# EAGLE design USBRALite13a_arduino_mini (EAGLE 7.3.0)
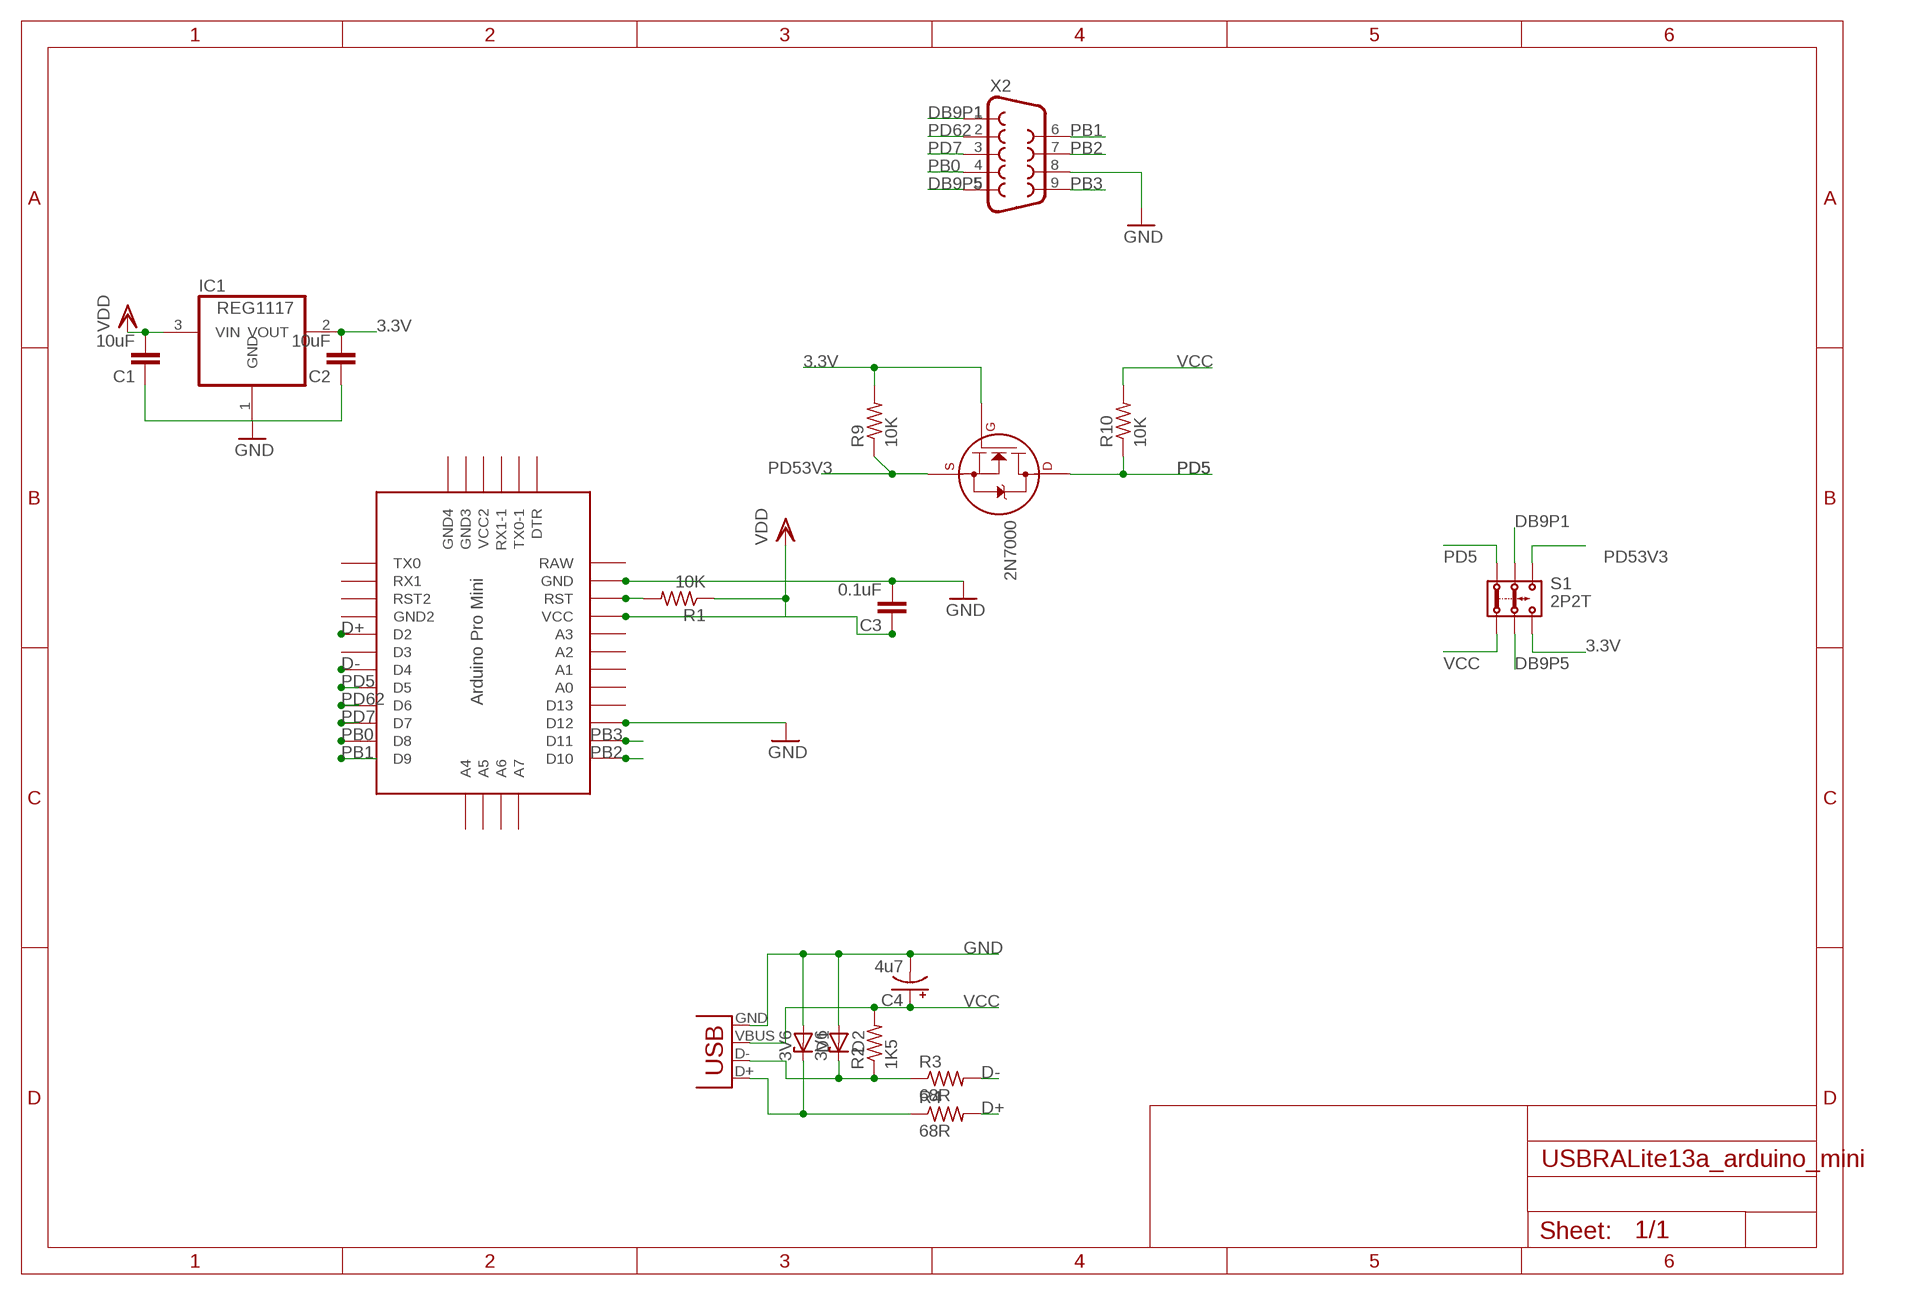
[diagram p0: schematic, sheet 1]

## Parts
2N7000  2N7000_TO92  [TO-92]
C1  10uF  C-EU050-024X044  [C050-024X044]
C2  10uF  C-EU050-024X044  [C050-024X044]
C3  0.1uF  C-EU050-024X044  [C050-024X044]
C4  4u7  CPOL-USE2.5-6  [E2,5-6]
D1  3V6  ZENER-DIODEZD-5  [ZDIO-5]
D2  3V6  ZENER-DIODEZD-5  [ZDIO-5]
IC1  REG1117  [SOT223]
R1  10K  R-US_0207/10  [0207/10]
R2  1K5  R-US_0207/10  [0207/10]
R3  68R  R-US_0207/10  [0207/10]
R4  68R  R-US_0207/10  [0207/10]
R9  10K  R-US_0207/10  [0207/10]
R10  10K  R-US_0207/10  [0207/10]
S1  2P2T  [2P2T]
U$1  PRO-MINI  [PRO-MINI]
X1  USBPTH  [USB-B-PTH]
X2  DB9MALE  [DB9_MALE]

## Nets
3.3V: 2N7000.2(G) C2.2 IC1.2(VOUT) R9.2 S1.3.2
D+: R4.2 U$1.D2
D-: R3.2 U$1.D4
DB9P1: S1.2.1 X2.1
DB9P5: S1.2.2 X2.5
GND: C1.1 C2.1 C3.2 C4.- D1.A D2.A IC1.1(GND) U$1.D12 U$1.GND X1.GND X2.8
N$1: R1.2 U$1.RST
N$8: D1.C R4.1 X1.D+
N$9: D2.C R2.1 R3.1 X1.D-
PB0: U$1.D8 X2.4
PB1: U$1.D9 X2.6
PB2: U$1.D10 X2.7
PB3: U$1.D11 X2.9
PD5: 2N7000.3(D) R10.1 S1.1.1 U$1.D5
PD7: U$1.D7 X2.3
PD53V3: 2N7000.1(S) R9.1 S1.3.1
PD62: U$1.D6 X2.2
VCC: C3.1 C4.+ R1.1 R2.2 R10.2 S1.1.2 X1.VBUS ; supply symbol labelled VDD
VDD: C1.2 IC1.3(VIN)
Unconnected: U$1.A0 U$1.A1 U$1.A2 U$1.A3 U$1.A4 U$1.A5 U$1.A6 U$1.A7 U$1.D3 U$1.D13 U$1.DTR U$1.GND1(GND2) U$1.GND2(GND4) U$1.GND3 U$1.RST1(RST2) U$1.RX1 U$1.RX1-1 U$1.TX0 U$1.TX0-1 U$1.VCC U$1.VCC1(VCC2)

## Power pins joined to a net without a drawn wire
RAW: U$1.RAW

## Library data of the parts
2N7000 = transistors:2N700*: 2N7000, 2N7002, NDS7002A N-channel enhancement mode MOSFET
C1-C3 = rcl:C-EU: CAPACITOR, European symbol
C4 = adafruit:CPOL-US: POLARIZED CAPACITOR, American symbol
D1 D2 = diode:ZENER-DIODE: Z-Diode
IC1 = burr-brown:REG1117: 800mA and 1A Low Dropout (LDO) Positive Regulator 1.8V, 2.5V, 2.85V, 3.3V, 5V, and Adj; MPN: REG1117; OC_FARNELL: 1097566; OC_NEWARK: 14P6981
R1-R4 R9 R10 = adafruit:R-US_: RESISTOR, American symbol
S1 = Itead_BP_110825:2P2T: BAS011
U$1 = Arduino-clone:PRO-MINI: Arduion Pro Mini Clone V1.0 www.betemcu.cu
X1 = SparkFun:USB: USB Connectors USB-B-PTH is fully proven SKU : PRT-00139 USB-miniB is fully proven SKU : PRT-00587 USB-A-PCB is untested. USB-A-H is throughly reviewed, but untested. Spark Fun Electronics SKU : PRT-00437 USB-B-SMT is throughly reviewed, but untested. Needs silkscreen touching up. USB-A-S has not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
X2 = SparkFun:DB9: DB9 Connector Standard DB9 (D-Sub 9) serial connector. Can be used for CAN bus as well as RS485 and RS232. Footprint production proven. Spark Fun Electronics SKU : PRT-00429

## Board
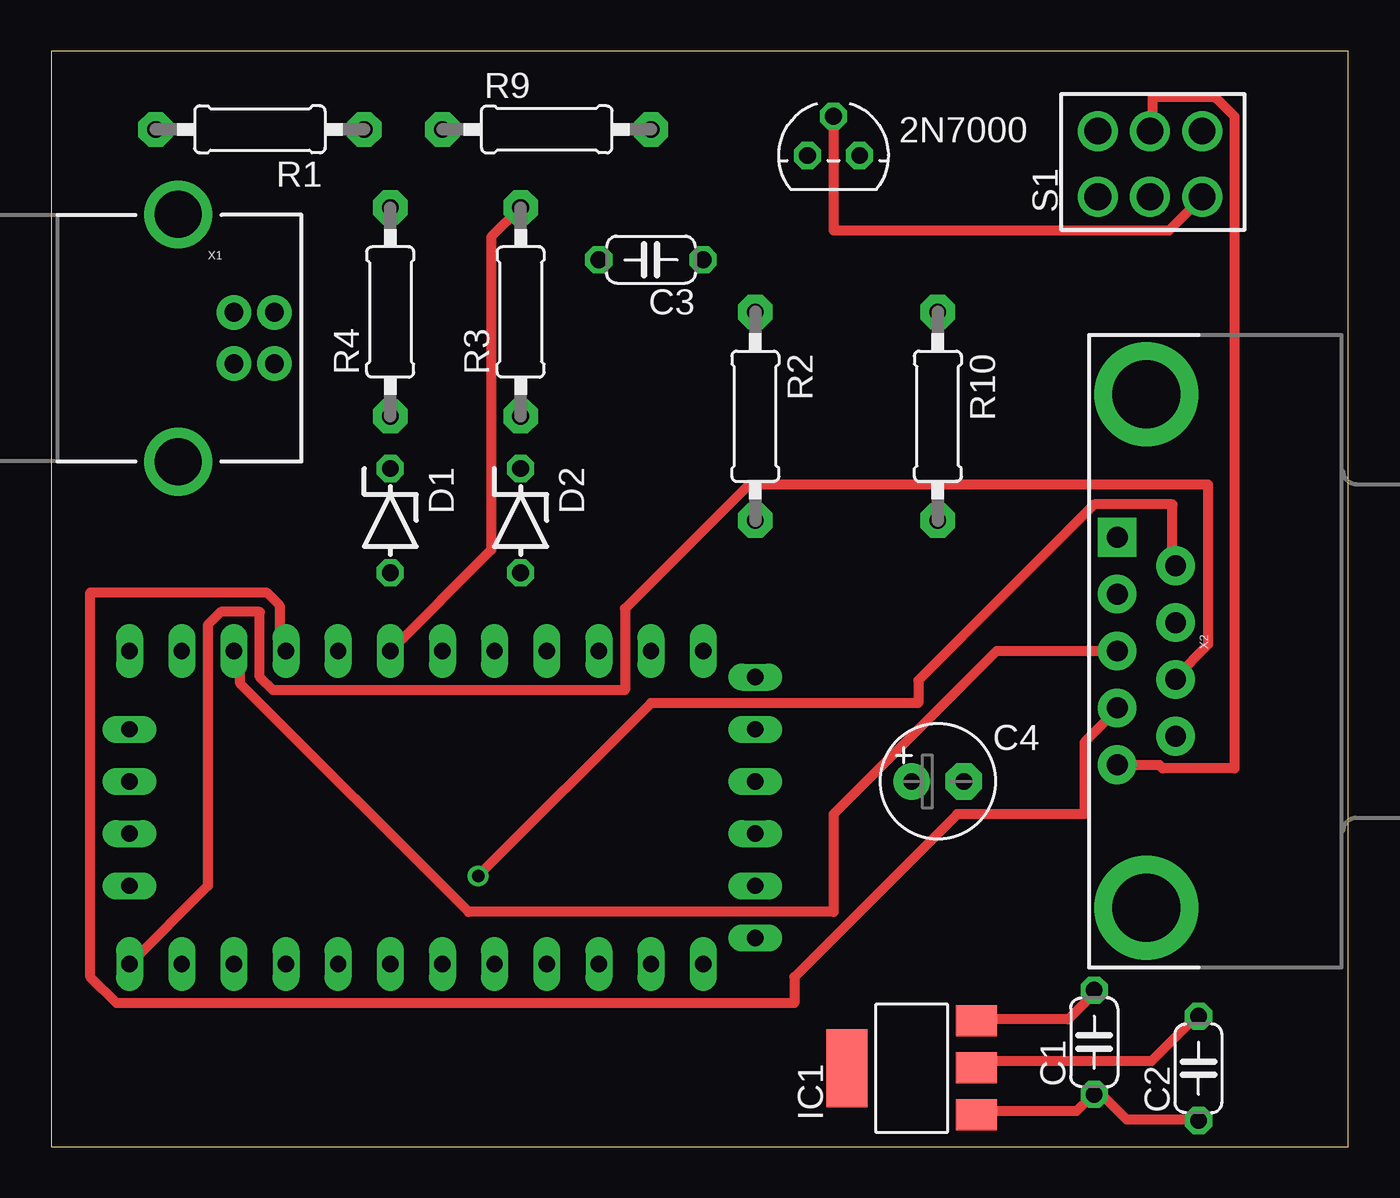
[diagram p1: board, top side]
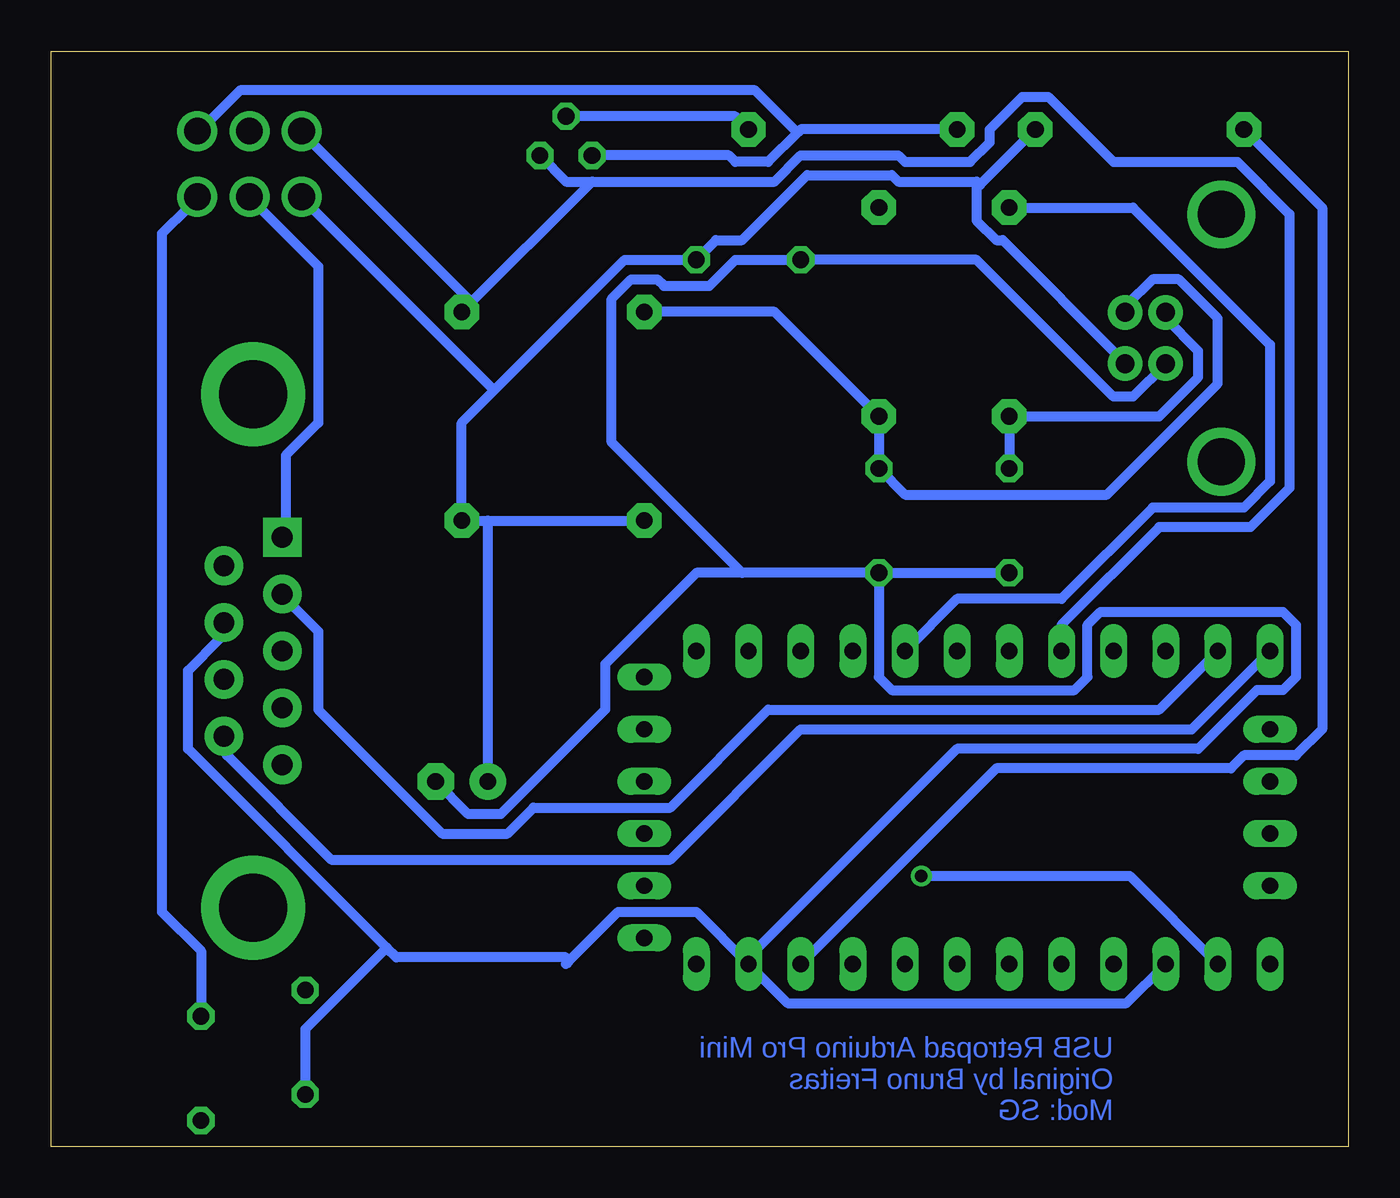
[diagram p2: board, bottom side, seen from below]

Size 63.17 x 53.33 mm. Coordinates in mm from the lower left corner, seen from the top.
Outline: 0,0 63.17,0 63.17,53.33 0,53.33 0,0
Copper layers (1*16): Top 0.035mm / dielectric 1.5mm / Bottom 0.035mm
Design rules "default *": minimum track width 19mil, minimum drill 24mil, track to track 13mil, track to pad 13mil, pad to pad 13mil, via to via 13mil, smd to smd 13mil, copper to edge 40mil, drill to drill 8mil, minimum pad ring 10mil, minimum via ring 8mil, stop-mask expansion 4mil, vias tented up to drill 0mil, thermal gap 10mil

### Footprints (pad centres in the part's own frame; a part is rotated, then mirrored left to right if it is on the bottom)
TO-92 = drill 0.813 octagon: 1 -1.27,0; 2 0,1.905; 3 1.27,0
C050-024X044 = drill 0.813 octagon: 1 -2.54,0; 2 2.54,0
E2,5-6 = drill 0.813 pad 1.778: + -1.27,0 | drill 0.813 pad 1.778 octagon: - 1.27,0
ZDIO-5 = drill 0.813 octagon: A 2.54,0; C -2.54,0
SOT223 = smd 1.499 x 2.007: 1 -2.261,-3.15; 2 0.025,-3.15; 3 2.311,-3.15 | smd 3.81 x 2.007: 4 0,3.15
0207/10 = drill 0.813 pad 1.676 octagon: 1 -5.08,0; 2 5.08,0
2P2T = drill 1.3 pad 1.93: 1.1 -3.635,-0.085; 1.2 -3.635,-3.285; 2.1 -1.095,-0.085; 2.2 -1.095,-3.285; 3.1 1.445,-0.085; 3.2 1.445,-3.285
PRO-MINI = drill 0.8 long: A0 8.89,8.89; A1 8.89,11.43; A2 8.89,13.97; A3 8.89,16.51; A4 -2.54,-1.27; A5 0,-1.27; A6 2.54,-1.27; A7 5.08,-1.27; D2 -6.35,16.51; D3 -6.35,13.97; D4 -6.35,11.43; D5 -6.35,8.89; D6 -6.35,6.35; D7 -6.35,3.81; D8 -6.35,1.27; D9 -6.35,-1.27; D10 8.89,-1.27; D11 8.89,1.27; D12 8.89,3.81; D13 8.89,6.35; DTR 7.62,29.21; GND 8.89,24.13; GND1 -6.35,19.05; GND2 -5.08,29.21; GND3 -2.54,29.21; RAW 8.89,26.67; RST 8.89,21.59; RST1 -6.35,21.59; RX1 -6.35,24.13; RX1-1 2.54,29.21; TX0 -6.35,26.67; TX0-1 5.08,29.21; VCC 8.89,19.05; VCC1 0,29.21
USB-B-PTH = drill 0.914 pad 1.676: D+ 0,1.25; D- 1.981,1.25; GND 0,-1.25; VBUS 1.981,-1.25 | drill 2.286: S1 -2.718,-6.02; S2 -2.718,6.02
DB9_MALE = drill 1.016 pad 1.88: 1 5.54,-1.42; 2 2.77,-1.42; 3 0,-1.42; 4 -2.77,-1.42; 6 4.15,1.42; 7 1.38,1.42; 8 -1.38,1.42; 9 -4.15,1.42 | drill 1.016 pad 1.88 square: 5 -5.54,-1.42 | drill 3.302 pad 5.08: G1 -12.5,0; G2 12.5,0

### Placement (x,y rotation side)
2N7000  38.1,48.26 0 top
C1  50.8,5.08 90 top
C2  55.88,3.81 90 top
C3  29.21,43.18 180 top
C4  43.18,17.78 0 top
D1  16.51,30.48 270 top
D2  22.86,30.48 270 top
IC1  41.91,3.81 90 top
R1  10.16,49.53 180 top
R2  34.29,35.56 270 top
R3  22.86,40.64 90 top
R4  16.51,40.64 90 top
R9  24.13,49.53 0 top
R10  43.18,35.56 270 top
S1  54.61,49.53 0 top
U$1  5.08,17.78 270 top
X1  8.89,39.37 0 top
X2  53.34,24.13 270 top

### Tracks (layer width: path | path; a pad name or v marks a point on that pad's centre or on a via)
3.3V
  Top 0.483: 2N7000.2 38.1,44.61 54.45,44.61 56.04,46.2 S1.3.2 | IC1.2 45.06,4.17 53.59,4.17 55.63,6.2 C2.2
  Bottom 0.483: 2N7000.2 29.84,50.17 R9.2 | C2.2 55.88,9.53 57.78,11.43 57.78,44.45 56.51,45.72 S1.3.2
D+
  Bottom 0.483: U$1.D2 19.05,26.67 13.97,26.67 9.53,31.11 5.08,31.11 3.81,32.39 3.81,39.05 10.48,45.72 R4.2
D-
  Top 0.483: U$1.D4 21.43,29.05 21.43,44.29 R3.2
DB9P1
  Top 0.483: X2.1 52.07,18.57 53.97,18.57 54.13,18.41 57.63,18.41 57.63,50.17 56.67,51.12 53.66,51.12 53.66,49.53 S1.2.1
DB9P5
  Bottom 0.483: X2.5 51.75,29.84 51.75,33.66 50.16,35.24 50.16,42.86 53.34,46.04 S1.2.2
GND
  Top 0.483: IC1.1 45.06,1.73 49.94,1.73 50.75,2.54 C1.1 51.16,2.54 52.38,1.32 55.63,1.32 C2.1
  Bottom 0.483: U$1.GND 31.75,11.43 35.56,11.43 37.94,9.05 | 38.1,8.89 37.94,9.05 | 46.83,9.68 46.35,9.21 38.1,9.21 37.94,9.05 | 46.83,9.68 56.51,19.37 56.51,23.18 54.93,24.76 54.93,25.4 X2.8 | X1.GND 8.89,38.1 10.48,36.51 11.43,36.51 18.1,43.18 C3.2 29.84,43.18 31.11,41.91 33.34,41.91 33.65,42.23 34.92,42.23 35.88,41.28 35.88,34.29 29.53,27.94 | D2.A D1.A | C4.- 42.86,16.19 41.27,16.19 36.2,21.27 36.2,23.5 31.75,27.94 29.53,27.94 | D2.A 29.53,27.94 | D2.A 22.86,22.86 22.23,22.22 13.34,22.22 12.7,22.86 12.7,25.4 12.07,26.04 3.18,26.04 2.54,25.4 2.54,22.86 3.18,22.22 4.45,22.22 7.3,19.37 19.05,19.37 29.21,9.21 U$1.GND | U$1.D12 10.79,6.98 27.3,6.98 U$1.GND | C1.1 50.8,5.71 46.83,9.68
N$1
  Bottom 0.483: U$1.RST 17.14,18.41 5.71,18.41 5.08,19.05 2.54,19.05 1.27,20.32 1.27,45.72 R1.2
N$8
  Bottom 0.483: D1.C R4.1 9.21,35.56 7.3,37.47 7.3,38.73 8.89,40.32 X1.D+
N$9
  Bottom 0.483: X1.D- 10.79,40.64 10.79,40.96 9.53,42.23 8.26,42.23 6.35,40.32 6.35,37.15 11.75,31.75 21.59,31.75 D2.C R3.1 27.94,40.64 R2.1
PB0
  Bottom 0.483: U$1.D8 9.21,21.27 28.26,21.27 33.02,16.51 39.69,16.51 40.96,15.24 44.13,15.24 50.16,21.27 50.16,25.08 51.75,26.67 X2.4
PB1
  Bottom 0.483: U$1.D9 7.62,20.32 26.67,20.32 33.02,13.97 49.53,13.97 54.61,19.05 54.61,19.68 X2.6
PB2
  Top 0.483: U$1.D10 7.62,12.7 7.62,25.4 8.26,26.04 10.16,26.04 10.16,22.86 10.79,22.22 27.94,22.22 27.94,26.19 33.97,32.23 56.36,32.23 56.36,24.45 54.77,22.86 X2.7
PB3  (via drill 0.61)
  Top 0.483: v20.8,13.18 29.21,21.59 42.23,21.59 42.23,22.7 50.8,31.27 54.61,31.27 54.61,28.42 X2.9
  Bottom 0.483: U$1.D11 10.64,13.18 v20.8,13.18
PD5
  Bottom 0.483: U$1.D5 13.97,25.4 9.21,30.16 4.76,30.16 2.86,32.07 2.86,45.4 5.4,47.94 11.43,47.94 14.61,51.12 15.88,51.12 17.46,49.53 17.46,48.89 18.41,47.94 21.59,47.94 21.91,48.26 26.67,48.26 27.94,46.99 36.83,46.99 | 36.83,46.99 38.1,46.99 2N7000.3 | 36.83,46.99 R10.1 42.86,41.28 50.8,49.21 S1.1.1
PD7
  Top 0.483: U$1.D7 9.21,23.81 9.21,22.54 20.32,11.43 38.1,11.43 38.1,16.19 46.04,24.13 X2.3
PD53V3
  Bottom 0.483: 2N7000.1 30.16,48.26 29.84,47.94 28.26,47.94 26.83,49.37 | 26.83,49.37 26.67,49.53 R9.1 | 26.83,49.37 28.89,51.44 53.97,51.44 55.88,49.53 S1.3.1
PD62
  Top 0.483: U$1.D6 11.11,24.45 11.11,26.35 10.48,26.99 1.9,26.99 1.9,8.25 3.18,6.98 36.2,6.98 36.2,8.25 44.13,16.19 50.32,16.19 50.32,19.68 51.91,21.27 X2.2
VCC
  Bottom 0.483: R1.1 17.94,46.83 | 17.94,46.83 18.1,46.67 18.1,45.09 17.14,44.13 16.83,44.13 11.11,38.42 X1.VBUS | 41.59,36.83 43.18,35.24 R10.2 41.91,30.48 | 41.59,36.83 35.24,43.18 C3.1 30.8,44.13 29.53,44.13 26.35,47.31 22.23,47.31 21.91,46.99 18.1,46.99 17.94,46.83 | 41.91,30.48 R2.2 | 41.91,30.48 C4.+ | 41.59,36.83 50.8,46.04 S1.1.2
VDD
  Top 0.483: IC1.3 45.06,6.2 49.53,6.2 50.75,7.42 C1.2

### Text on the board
Bottom: USB Retropad Arduino Pro Mini / Original by Bruno Freitas / Mod: SG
